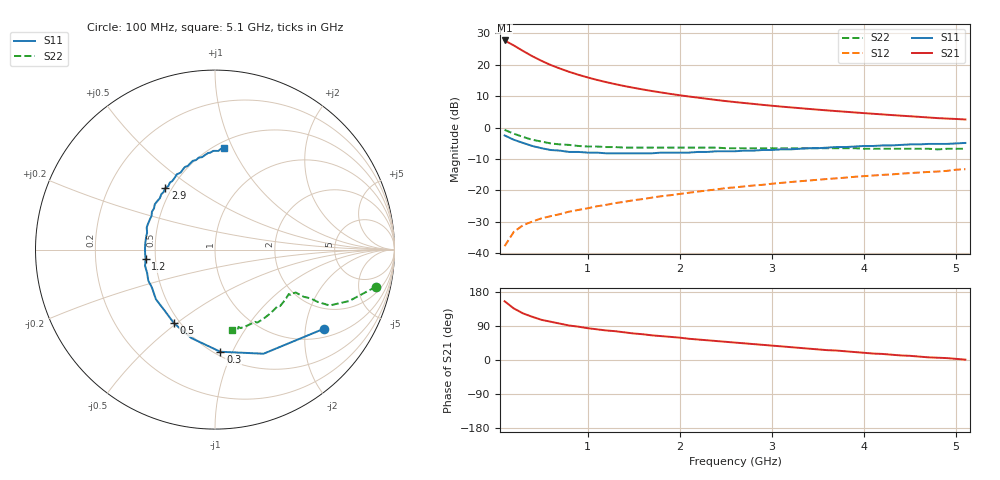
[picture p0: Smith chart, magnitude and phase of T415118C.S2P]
!AT-41511
!S AND NOISE PARAMETERS at Vce=8V  Ic=10mA.  LAST UPDATED 08-03-92
# ghz s ma r 50
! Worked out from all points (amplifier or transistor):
!   51 points, 100 MHz to 5.1 GHz, reference 50 ohm
!   highest |S21| = 27.7 dB at 100 MHz (marker M1)
!   |S21| within 3 dB of that: start of sweep to 280.3 MHz
!   unconditionally stable (mu >= 1): 1.177 GHz to 3.393 GHz; 3.465 GHz to 3.503 GHz
!   at 900 MHz: K = 0.90, MSG = 21.5 dB, |S12| = -26.2 dB
!   at 2.6 GHz: K = 1.07, MAG = 11.9 dB, |S12| = -19.0 dB
!   at 5.1 GHz: K = 0.85, MSG = 7.9 dB, |S12| = -13.2 dB
!   lowest NFmin = 1.10 dB at 100 MHz
!   S11 on the Smith chart (normalised r, x): 100 MHz: 1.25, -2.53; 300 MHz: 0.53, -0.90; 500 MHz: 0.46, -0.49; 1.2 GHz: 0.44, -0.06; 2.9 GHz: 0.46, +0.39; 5.1 GHz: 0.55, +0.93
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0.1  0.75 -36.0  24.3 155.0  0.013 73.0  0.92 -13.0
0.2  0.64 -65.0  20.24 136.0  0.022 62.0  0.8 -21.0
0.3  0.57 -87.0  16.53 123.0  0.028 57.0  0.71 -26.0
0.4  0.51 -105.0  13.67 114.0  0.032 54.0  0.64 -27.0
0.5  0.47 -119.0  11.54 106.0  0.036 53.0  0.6 -27.0
0.6  0.44 -130.0  9.897 101.0  0.039 53.0  0.56 -28.0
0.7  0.43 -140.0  8.691 96.0  0.042 54.0  0.54 -28.0
0.8  0.41 -149.0  7.709 91.0  0.046 55.0  0.53 -28.0
0.9  0.41 -155.0  6.921 88.0  0.049 55.0  0.51 -28.0
1  0.4 -161.0  6.281 84.0  0.052 56.0  0.5 -29.0
1.1  0.4 -167.0  5.74 81.0  0.056 57.0  0.5 -29.0
1.2  0.39 -172.0  5.295 78.0  0.059 57.0  0.49 -30.0
1.4  0.39 178.0  4.577 73.0  0.066 58.0  0.48 -31.0
1.5  0.39 174.0  4.294 70.0  0.07 58.0  0.48 -32.0
1.7  0.39 166.0  3.813 65.0  0.077 59.0  0.48 -34.0
1.8  0.4 162.0  3.615 63.0  0.081 59.0  0.48 -35.0
2.1  0.4 152.0  3.121 56.0  0.092 58.0  0.48 -38.0
2.6  0.42 137.0  2.546 46.0  0.112 57.0  0.47 -43.0
2.9  0.44 129.0  2.298 40.0  0.123 56.0  0.47 -47.0
3.5  0.47 114.0  1.927 28.0  0.148 53.0  0.47 -54.0
4.3  0.52 98.0  1.582 14.0  0.18 48.0  0.46 -65.0
5.1  0.57 85.0  1.346 1.0  0.218 44.0  0.46 -78.0
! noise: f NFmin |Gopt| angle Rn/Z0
0.1  1.1  0.4  6  0.27
0.9  1.3  0.33  62  0.2
1.8  1.6  0.27  135  0.13
2.4  1.8  0.35  178  0.1
